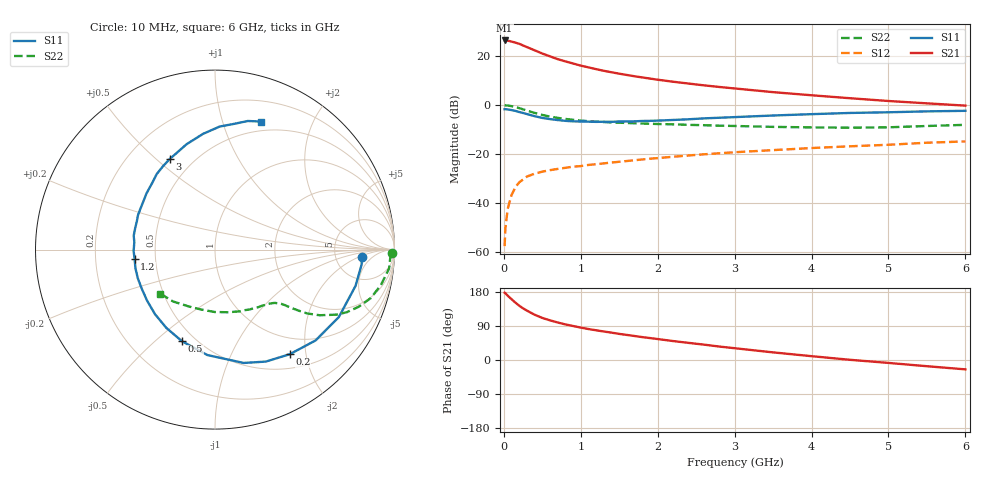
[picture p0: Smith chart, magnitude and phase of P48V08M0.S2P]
! SIEMENS Small Signal Semiconductors
! BFP182
! Si NPN RF Bipolar Junction Transistor in SOT143
! VCE = 8 V  IC = 8 mA
! Common Emitter S-Parameters:  March  1996
# GHz  S  MA  R  50
!  f  S11  S21  S12  S22
! GHz  MAG  ANG  MAG  ANG  MAG  ANG  MAG  ANG
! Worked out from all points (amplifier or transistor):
!   36 points, 10 MHz to 6 GHz, reference 50 ohm
!   highest |S21| = 26.4 dB at 10 MHz (marker M1)
!   |S21| within 3 dB of that: start of sweep to 322.1 MHz
!   unconditionally stable (mu >= 1): 1.392 GHz to 5.61 GHz
!   at 250 MHz: K = 0.27, MSG = 27.4 dB, |S12| = -30.5 dB
!   at 1.4 GHz: K = 1.00, MAG = 18.1 dB, |S12| = -23.5 dB
!   at 6 GHz: K = 0.97, MSG = 7.3 dB, |S12| = -14.9 dB
!   lowest NFmin = 1.40 dB at 450 MHz
!   S11 on the Smith chart (normalised r, x): 10 MHz: 9.49, -2.40; 200 MHz: 0.72, -1.71; 500 MHz: 0.42, -0.62; 1.2 GHz: 0.38, -0.05; 3 GHz: 0.37, +0.55; 6 GHz: 0.40, +1.34
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0.01  0.8199 -2.9  20.79 177.6  0.0013 91.1  0.984 -1.2
0.02  0.8212 -5.8  20.7 176.1  0.003 87.1  0.9779 -2.4
0.05  0.8087 -14.5  20.57 169.8  0.0075 86.5  0.9756 -6.2
0.1  0.7858 -28.6  19.75 160.4  0.0144 74.9  0.9451 -12.1
0.15  0.7551 -42.1  18.77 151.5  0.0208 69.0  0.909 -17.3
0.2  0.7162 -54.5  17.78 143.3  0.0262 63.7  0.8616 -21.7
0.25  0.6852 -65.6  16.42 136.2  0.0299 58.8  0.8131 -25.4
0.3  0.6515 -75.8  15.22 130.4  0.0344 55.4  0.7671 -28.2
0.4  0.5892 -94.1  13.07 119.4  0.0394 49.8  0.6883 -32.1
0.5  0.5429 -109.7  11.23 111.1  0.0433 45.7  0.625 -34.7
0.6  0.5138 -121.8  9.849 104.6  0.0465 44.1  0.5775 -36.1
0.7  0.4911 -132.9  8.626 99.0  0.0493 42.7  0.5444 -37.1
0.8  0.4733 -143.1  7.771 93.9  0.0519 41.8  0.5179 -37.9
1.1  0.4552 -166.9  5.857 81.7  0.0594 41.2  0.4665 -40.0
1.2  0.4508 -173.6  5.389 78.4  0.0616 40.7  0.4557 -40.9
1.7  0.4628 160.3  3.852 63.3  0.0742 40.7  0.4223 -46.0
2.2  0.4933 140.8  2.982 50.0  0.0873 39.2  0.4014 -53.1
3  0.5641 116.6  2.173 31.1  0.108 34.9  0.3719 -67.6
3.5  0.6085 105.0  1.827 20.1  0.1194 31.7  0.3563 -78.4
4.5  0.6862 87.8  1.372 0.5  0.1429 25.0  0.3427 -103.2
5.5  0.7394 75.7  1.078 -16.4  0.1691 18.6  0.3714 -128.9
6  0.7585 70.2  0.968 -24.7  0.1797 14.3  0.3921 -141.4
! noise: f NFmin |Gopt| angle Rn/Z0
0.45  1.4  0.26  41  0.29
0.9  1.5  0.25  83  0.23
1.8  2  0.21  162  0.2
